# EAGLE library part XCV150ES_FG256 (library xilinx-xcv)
xcv150es_fg256 edit this description Auto generated by make-symbol-device-package-bsdl.ulp Rev. 26 Source: xcv150es_fg256.bsd
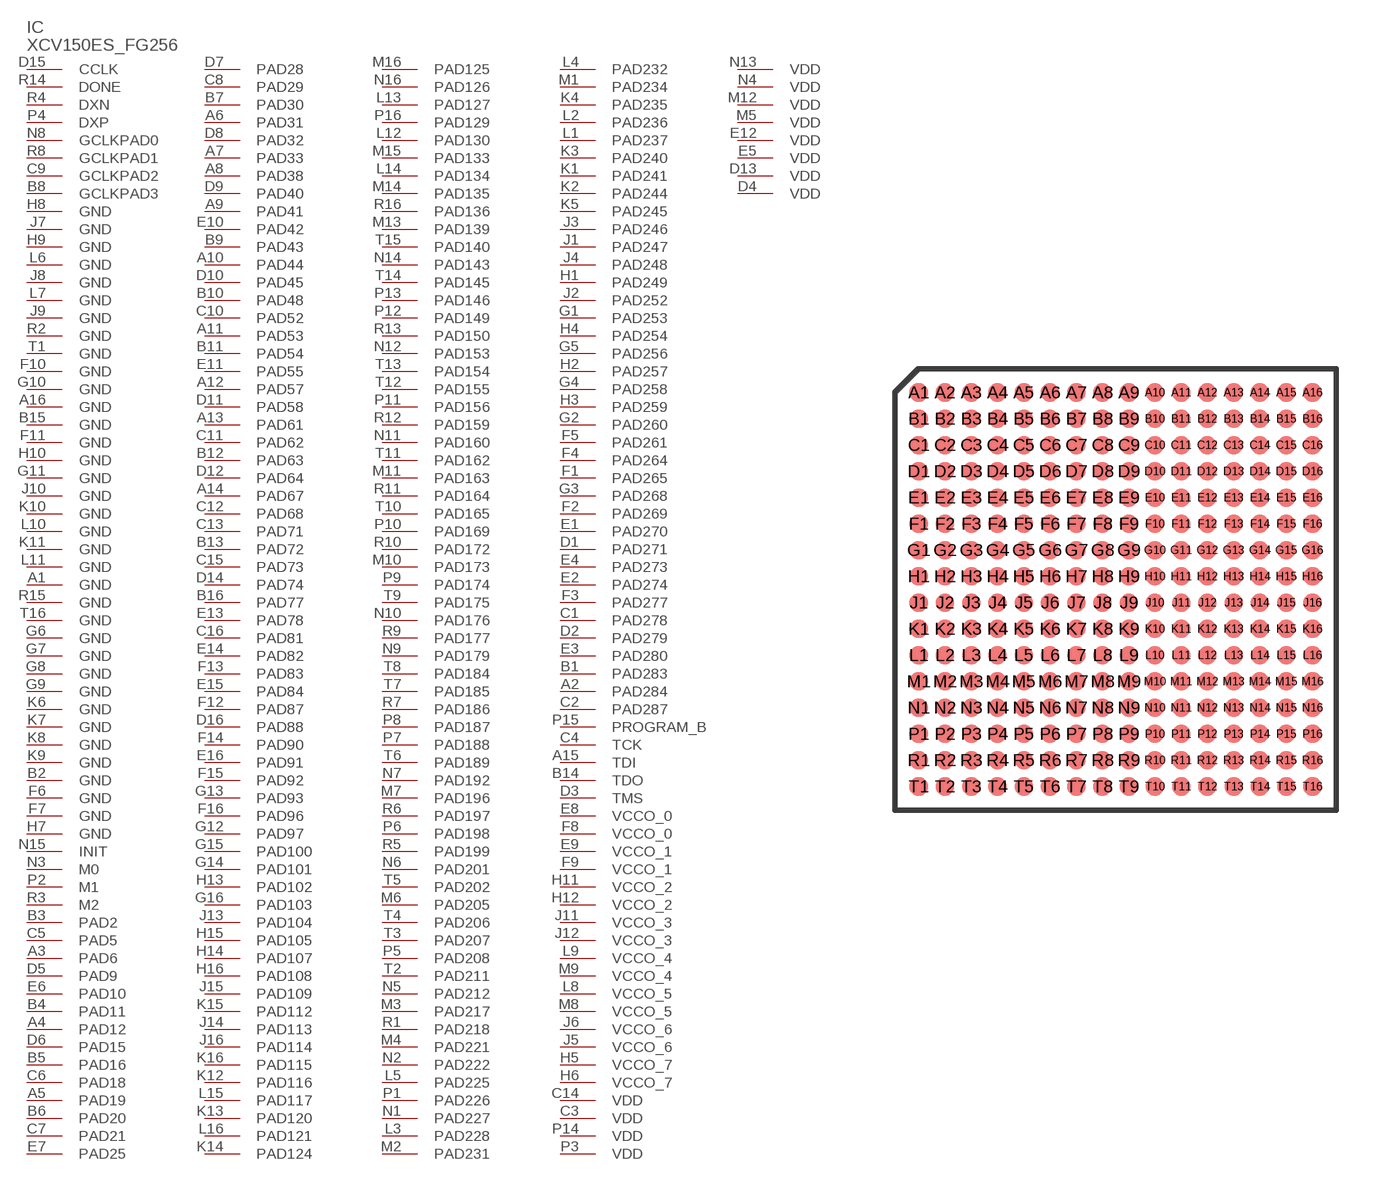
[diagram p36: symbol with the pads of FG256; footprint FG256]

Designator prefix IC

## XCV150ES_FG256 (OC_FARNELL: unknown; OC_NEWARK: unknown)  [FG256]
A1  GND  pwr
A2  PAD284
A3  PAD6
A4  PAD12
A5  PAD19
A6  PAD31
A7  PAD33
A8  PAD38
A9  PAD41
A10  PAD44
A11  PAD53
A12  PAD57
A13  PAD61
A14  PAD67
A15  TDI  in
A16  GND  pwr
B1  PAD283
B2  GND  pwr
B3  PAD2
B4  PAD11
B5  PAD16
B6  PAD20
B7  PAD30
B8  GCLKPAD3  in
B9  PAD43
B10  PAD48
B11  PAD54
B12  PAD63
B13  PAD72
B14  TDO  out
B15  GND  pwr
B16  PAD77
C1  PAD278
C2  PAD287
C3  VDD  pwr
C4  TCK  in
C5  PAD5
C6  PAD18
C7  PAD21
C8  PAD29
C9  GCLKPAD2  in
C10  PAD52
C11  PAD62
C12  PAD68
C13  PAD71
C14  VDD  pwr
C15  PAD73
C16  PAD81
D1  PAD271
D2  PAD279
D3  TMS  in
D4  VDD  pwr
D5  PAD9
D6  PAD15
D7  PAD28
D8  PAD32
D9  PAD40
D10  PAD45
D11  PAD58
D12  PAD64
D13  VDD  pwr
D14  PAD74
D15  CCLK
D16  PAD88
E1  PAD270
E2  PAD274
E3  PAD280
E4  PAD273
E5  VDD  pwr
E6  PAD10
E7  PAD25
E8  VCCO_0  pwr
E9  VCCO_1  pwr
E10  PAD42
E11  PAD55
E12  VDD  pwr
E13  PAD78
E14  PAD82
E15  PAD84
E16  PAD91
F1  PAD265
F2  PAD269
F3  PAD277
F4  PAD264
F5  PAD261
F6  GND  pwr
F7  GND  pwr
F8  VCCO_0  pwr
F9  VCCO_1  pwr
F10  GND  pwr
F11  GND  pwr
F12  PAD87
F13  PAD83
F14  PAD90
F15  PAD92
F16  PAD96
G1  PAD253
G2  PAD260
G3  PAD268
G4  PAD258
G5  PAD256
G6  GND  pwr
G7  GND  pwr
G8  GND  pwr
G9  GND  pwr
G10  GND  pwr
G11  GND  pwr
G12  PAD97
G13  PAD93
G14  PAD101
G15  PAD100
G16  PAD103
H1  PAD249
H2  PAD257
H3  PAD259
H4  PAD254
H5  VCCO_7  pwr
H6  VCCO_7  pwr
H7  GND  pwr
H8  GND  pwr
H9  GND  pwr
H10  GND  pwr
H11  VCCO_2  pwr
H12  VCCO_2  pwr
H13  PAD102
H14  PAD107
H15  PAD105
H16  PAD108
J1  PAD247
J2  PAD252
J3  PAD246
J4  PAD248
J5  VCCO_6  pwr
J6  VCCO_6  pwr
J7  GND  pwr
J8  GND  pwr
J9  GND  pwr
J10  GND  pwr
J11  VCCO_3  pwr
J12  VCCO_3  pwr
J13  PAD104
J14  PAD113
J15  PAD109
J16  PAD114
K1  PAD241
K2  PAD244
K3  PAD240
K4  PAD235
K5  PAD245
K6  GND  pwr
K7  GND  pwr
K8  GND  pwr
K9  GND  pwr
K10  GND  pwr
K11  GND  pwr
K12  PAD116
K13  PAD120
K14  PAD124
K15  PAD112
K16  PAD115
L1  PAD237
L2  PAD236
L3  PAD228
L4  PAD232
L5  PAD225
L6  GND  pwr
L7  GND  pwr
L8  VCCO_5  pwr
L9  VCCO_4  pwr
L10  GND  pwr
L11  GND  pwr
L12  PAD130
L13  PAD127
L14  PAD134
L15  PAD117
L16  PAD121
M1  PAD234
M2  PAD231
M3  PAD217
M4  PAD221
M5  VDD  pwr
M6  PAD205
M7  PAD196
M8  VCCO_5  pwr
M9  VCCO_4  pwr
M10  PAD173
M11  PAD163
M12  VDD  pwr
M13  PAD139
M14  PAD135
M15  PAD133
M16  PAD125
N1  PAD227
N2  PAD222
N3  M0  in
N4  VDD  pwr
N5  PAD212
N6  PAD201
N7  PAD192
N8  GCLKPAD0  in
N9  PAD179
N10  PAD176
N11  PAD160
N12  PAD153
N13  VDD  pwr
N14  PAD143
N15  INIT
N16  PAD126
P1  PAD226
P2  M1  in
P3  VDD  pwr
P4  DXP  pas
P5  PAD208
P6  PAD198
P7  PAD188
P8  PAD187
P9  PAD174
P10  PAD169
P11  PAD156
P12  PAD149
P13  PAD146
P14  VDD  pwr
P15  PROGRAM_B  in
P16  PAD129
R1  PAD218
R2  GND  pwr
R3  M2  in
R4  DXN  pas
R5  PAD199
R6  PAD197
R7  PAD186
R8  GCLKPAD1  in
R9  PAD177
R10  PAD172
R11  PAD164
R12  PAD159
R13  PAD150
R14  DONE
R15  GND  pwr
R16  PAD136
T1  GND  pwr
T2  PAD211
T3  PAD207
T4  PAD206
T5  PAD202
T6  PAD189
T7  PAD185
T8  PAD184
T9  PAD175
T10  PAD165
T11  PAD162
T12  PAD155
T13  PAD154
T14  PAD145
T15  PAD140
T16  GND  pwr

## Footprint FG256 (pad centres in mm)
Fine Pitch BGA (FG256) Auto generated by make-symbol-device-package-bsdl.ulp Rev. 26 Source: xcv100_fg256.bsd; fg256.pdf
smd 0.7 x 0.7: A1 -7.5,7.5; A2 -6.5,7.5; A3 -5.5,7.5; A4 -4.5,7.5; A5 -3.5,7.5; A6 -2.5,7.5; A7 -1.5,7.5; A8 -0.5,7.5; A9 0.5,7.5; A10 1.5,7.5; A11 2.5,7.5; A12 3.5,7.5; A13 4.5,7.5; A14 5.5,7.5; A15 6.5,7.5; A16 7.5,7.5; B1 -7.5,6.5; B2 -6.5,6.5; B3 -5.5,6.5; B4 -4.5,6.5; B5 -3.5,6.5; B6 -2.5,6.5; B7 -1.5,6.5; B8 -0.5,6.5; B9 0.5,6.5; B10 1.5,6.5; B11 2.5,6.5; B12 3.5,6.5; B13 4.5,6.5; B14 5.5,6.5; B15 6.5,6.5; B16 7.5,6.5; C1 -7.5,5.5; C2 -6.5,5.5; C3 -5.5,5.5; C4 -4.5,5.5; C5 -3.5,5.5; C6 -2.5,5.5; C7 -1.5,5.5; C8 -0.5,5.5; C9 0.5,5.5; C10 1.5,5.5; C11 2.5,5.5; C12 3.5,5.5; C13 4.5,5.5; C14 5.5,5.5; C15 6.5,5.5; C16 7.5,5.5; D1 -7.5,4.5; D2 -6.5,4.5; D3 -5.5,4.5; D4 -4.5,4.5; D5 -3.5,4.5; D6 -2.5,4.5; D7 -1.5,4.5; D8 -0.5,4.5; D9 0.5,4.5; D10 1.5,4.5; D11 2.5,4.5; D12 3.5,4.5; D13 4.5,4.5; D14 5.5,4.5; D15 6.5,4.5; D16 7.5,4.5; E1 -7.5,3.5; E2 -6.5,3.5; E3 -5.5,3.5; E4 -4.5,3.5; E5 -3.5,3.5; E6 -2.5,3.5; E7 -1.5,3.5; E8 -0.5,3.5; E9 0.5,3.5; E10 1.5,3.5; E11 2.5,3.5; E12 3.5,3.5; E13 4.5,3.5; E14 5.5,3.5; E15 6.5,3.5; E16 7.5,3.5; F1 -7.5,2.5; F2 -6.5,2.5; F3 -5.5,2.5; F4 -4.5,2.5; F5 -3.5,2.5; F6 -2.5,2.5; F7 -1.5,2.5; F8 -0.5,2.5; F9 0.5,2.5; F10 1.5,2.5; F11 2.5,2.5; F12 3.5,2.5; F13 4.5,2.5; F14 5.5,2.5; F15 6.5,2.5; F16 7.5,2.5; G1 -7.5,1.5; G2 -6.5,1.5; G3 -5.5,1.5; G4 -4.5,1.5; G5 -3.5,1.5; G6 -2.5,1.5; G7 -1.5,1.5; G8 -0.5,1.5; G9 0.5,1.5; G10 1.5,1.5; G11 2.5,1.5; G12 3.5,1.5; G13 4.5,1.5; G14 5.5,1.5; G15 6.5,1.5; G16 7.5,1.5; H1 -7.5,0.5; H2 -6.5,0.5; H3 -5.5,0.5; H4 -4.5,0.5; H5 -3.5,0.5; H6 -2.5,0.5; H7 -1.5,0.5; H8 -0.5,0.5; H9 0.5,0.5; H10 1.5,0.5; H11 2.5,0.5; H12 3.5,0.5; H13 4.5,0.5; H14 5.5,0.5; H15 6.5,0.5; H16 7.5,0.5; J1 -7.5,-0.5; J2 -6.5,-0.5; J3 -5.5,-0.5; J4 -4.5,-0.5; J5 -3.5,-0.5; J6 -2.5,-0.5; J7 -1.5,-0.5; J8 -0.5,-0.5; J9 0.5,-0.5; J10 1.5,-0.5; J11 2.5,-0.5; J12 3.5,-0.5; J13 4.5,-0.5; J14 5.5,-0.5; J15 6.5,-0.5; J16 7.5,-0.5; K1 -7.5,-1.5; K2 -6.5,-1.5; K3 -5.5,-1.5; K4 -4.5,-1.5; K5 -3.5,-1.5; K6 -2.5,-1.5; K7 -1.5,-1.5; K8 -0.5,-1.5; K9 0.5,-1.5; K10 1.5,-1.5; K11 2.5,-1.5; K12 3.5,-1.5; K13 4.5,-1.5; K14 5.5,-1.5; K15 6.5,-1.5; K16 7.5,-1.5; L1 -7.5,-2.5; L2 -6.5,-2.5; L3 -5.5,-2.5; L4 -4.5,-2.5; L5 -3.5,-2.5; L6 -2.5,-2.5; L7 -1.5,-2.5; L8 -0.5,-2.5; L9 0.5,-2.5; L10 1.5,-2.5; L11 2.5,-2.5; L12 3.5,-2.5; L13 4.5,-2.5; L14 5.5,-2.5; L15 6.5,-2.5; L16 7.5,-2.5; M1 -7.5,-3.5; M2 -6.5,-3.5; M3 -5.5,-3.5; M4 -4.5,-3.5; M5 -3.5,-3.5; M6 -2.5,-3.5; M7 -1.5,-3.5; M8 -0.5,-3.5; M9 0.5,-3.5; M10 1.5,-3.5; M11 2.5,-3.5; M12 3.5,-3.5; M13 4.5,-3.5; M14 5.5,-3.5; M15 6.5,-3.5; M16 7.5,-3.5; N1 -7.5,-4.5; N2 -6.5,-4.5; N3 -5.5,-4.5; N4 -4.5,-4.5; N5 -3.5,-4.5; N6 -2.5,-4.5; N7 -1.5,-4.5; N8 -0.5,-4.5; N9 0.5,-4.5; N10 1.5,-4.5; N11 2.5,-4.5; N12 3.5,-4.5; N13 4.5,-4.5; N14 5.5,-4.5; N15 6.5,-4.5; N16 7.5,-4.5; P1 -7.5,-5.5; P2 -6.5,-5.5; P3 -5.5,-5.5; P4 -4.5,-5.5; P5 -3.5,-5.5; P6 -2.5,-5.5; P7 -1.5,-5.5; P8 -0.5,-5.5; P9 0.5,-5.5; P10 1.5,-5.5; P11 2.5,-5.5; P12 3.5,-5.5; P13 4.5,-5.5; P14 5.5,-5.5; P15 6.5,-5.5; P16 7.5,-5.5; R1 -7.5,-6.5; R2 -6.5,-6.5; R3 -5.5,-6.5; R4 -4.5,-6.5; R5 -3.5,-6.5; R6 -2.5,-6.5; R7 -1.5,-6.5; R8 -0.5,-6.5; R9 0.5,-6.5; R10 1.5,-6.5; R11 2.5,-6.5; R12 3.5,-6.5; R13 4.5,-6.5; R14 5.5,-6.5; R15 6.5,-6.5; R16 7.5,-6.5; T1 -7.5,-7.5; T2 -6.5,-7.5; T3 -5.5,-7.5; T4 -4.5,-7.5; T5 -3.5,-7.5; T6 -2.5,-7.5; T7 -1.5,-7.5; T8 -0.5,-7.5; T9 0.5,-7.5; T10 1.5,-7.5; T11 2.5,-7.5; T12 3.5,-7.5; T13 4.5,-7.5; T14 5.5,-7.5; T15 6.5,-7.5; T16 7.5,-7.5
